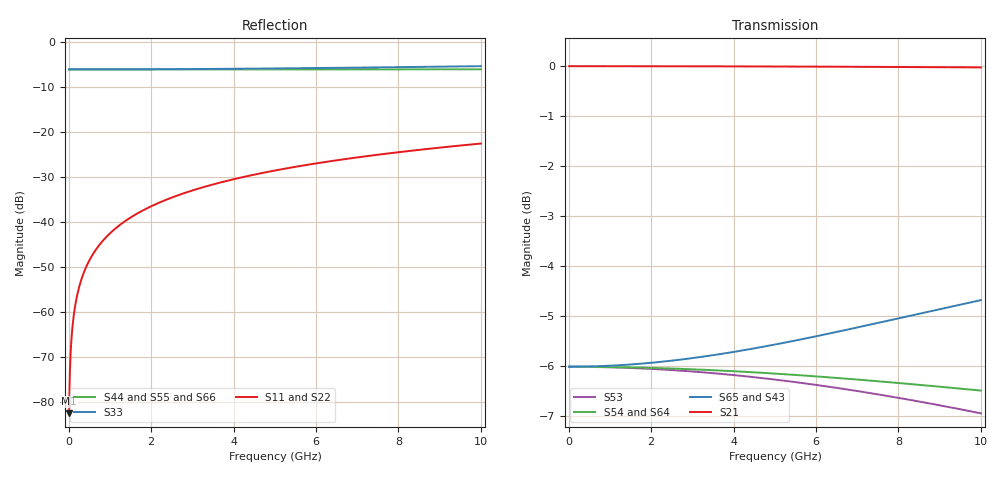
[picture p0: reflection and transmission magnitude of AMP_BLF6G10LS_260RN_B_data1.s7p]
! Created Thu Apr 01 01:00:00 2010
# ghz S ma R 50
! 7 Port Network Data from SP1.SP block
! freq  magS11  angS11  magS12  angS12  magS13  angS13  magS14  angS14
!  magS15  angS15  magS16  angS16  magS17  angS17
!  magS21  angS21
!  magS22  angS22  magS23  angS23  magS24  angS24  magS25  angS25
!  magS26  angS26  magS27  angS27
!  magS31  angS31  magS32  angS32
!  magS33  angS33  magS34  angS34  magS35  angS35  magS36  angS36
!  magS37  angS37
!  magS41  angS41  magS42  angS42  magS43  angS43
!  magS44  angS44  magS45  angS45  magS46  angS46  magS47  angS47
!  magS51  angS51  magS52  angS52  magS53  angS53  magS54  angS54
!  magS55  angS55  magS56  angS56  magS57  angS57
!  magS61  angS61
!  magS62  angS62  magS63  angS63  magS64  angS64  magS65  angS65
!  magS66  angS66  magS67  angS67
!  magS71  angS71  magS72  angS72
!  magS73  angS73  magS74  angS74  magS75  angS75  magS76  angS76
!  magS77  angS77
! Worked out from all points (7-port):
!   1000 points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, 10 MHz to 10 GHz, reference 50 ohm
!   strongest paths, dB at 10 MHz, 2.51 GHz, 5.01 GHz, 7.51 GHz, 10 GHz:
!     S21: 0.0, 0.0, 0.0, 0.0, 0.0
!     S65: -6.0, -5.9, -5.6, -5.1, -4.7
!     S43: -6.0, -5.9, -5.7, -5.4, -5.1
!     S54: -6.0, -6.1, -6.2, -6.3, -6.5
!     S64: -6.0, -6.1, -6.2, -6.4, -6.7
!     S53: -6.0, -6.1, -6.3, -6.6, -7.0
!   lowest |S11| = -82.5 dB at 10 MHz (marker M1), VSWR 1.00, Z = 50 + j0.00753 ohm
!   |S11| at or under -10 dB: start of sweep to end of sweep
